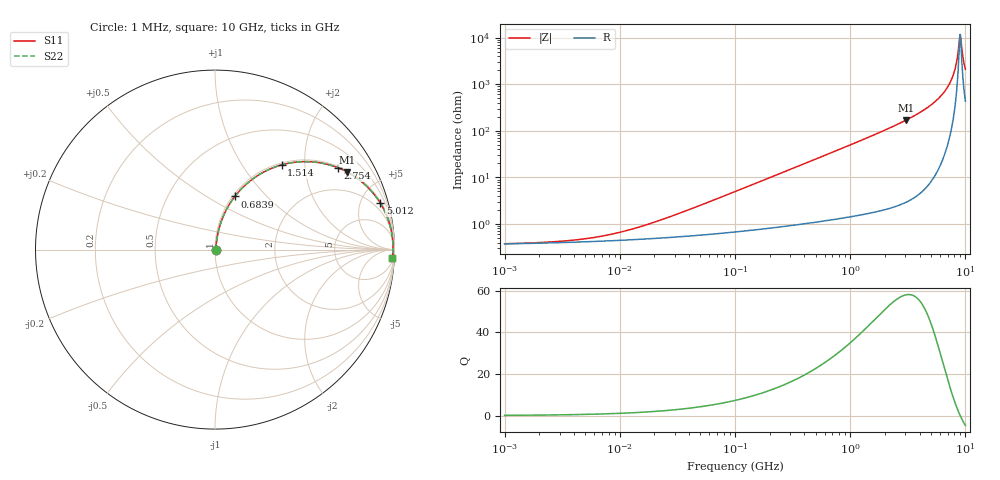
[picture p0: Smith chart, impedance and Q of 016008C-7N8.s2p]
# MHz S MA R 50
!Freq  MagS11  AngS11  MagS21  AngS21  MagS12  AngS12  MagS22  AngS22
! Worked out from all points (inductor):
!   801 points, 1 MHz to 10 GHz, reference 50 ohm
!   read as one part in series: L = 7.8 nH near 32.73 MHz
!   highest Q = 57.9 at 3.055 GHz (marker M1), where L = 8.81 nH
!   self-resonance near 8.913 GHz
!   S11 on the Smith chart (normalised r, x): 1 MHz: 1.01, +0.00; 683.9 MHz: 1.02, +0.67; 1.514 GHz: 1.03, +1.53; 2.754 GHz: 1.05, +2.98; 5.012 GHz: 1.16, +7.11; 10 GHz: 10, -41
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1  0.003751 7.5  0.9963 -0.0  0.9963 -0.0  0.003751 7.5
4.677351  0.004696 29.0  0.9959 -0.1  0.9959 -0.1  0.004696 29.0
9.772372  0.006503 46.9  0.9956 -0.3  0.9956 -0.3  0.006503 46.9
21.62719  0.01164 64.4  0.995 -0.6  0.995 -0.6  0.01164 64.4
101.1579  0.04964 79.4  0.9921 -2.8  0.9921 -2.8  0.04964 79.4
467.7351  0.222 74.5  0.9648 -12.8  0.9648 -12.8  0.222 74.5
683.9116  0.3162 69.5  0.9373 -18.4  0.9373 -18.4  0.3162 69.5
1023.293  0.448 61.8  0.8815 -26.6  0.8815 -26.6  0.448 61.8
1513.561  0.6003 51.8  0.7863 -36.9  0.7863 -36.9  0.6003 51.8
2162.719  0.7404 41.2  0.6582 -47.8  0.6582 -47.8  0.7404 41.2
2754.229  0.8235 33.6  0.553 -55.4  0.553 -55.4  0.8235 33.6
3054.921  0.8544 30.3  0.505 -58.7  0.505 -58.7  0.8544 30.3
5011.872  0.9571 15.6  0.2691 -73.1  0.2691 -73.1  0.9571 15.6
6237.348  0.9798 9.6  0.1671 -78.3  0.1671 -78.3  0.9798 9.6
7328.245  0.9889 5.4  0.09355 -80.5  0.09355 -80.5  0.9889 5.4
8035.261  0.9913 3.0  0.0522 -78.9  0.0522 -78.9  0.9913 3.0
8317.638  0.9916 2.1  0.03693 -75.9  0.03693 -75.9  0.9916 2.1
8709.636  0.9917 0.9  0.01745 -61.3  0.01745 -61.3  0.9917 0.9
8912.509  0.9916 0.3  0.009821 -31.0  0.009821 -31.0  0.9916 0.3
9225.714  0.9912 -0.6  0.01361 49.2  0.01361 49.2  0.9912 -0.6
9772.372  0.9898 -2.1  0.03741 73.2  0.03741 73.2  0.9898 -2.1
10000  0.9891 -2.7  0.04752 75.4  0.04752 75.4  0.9891 -2.7
